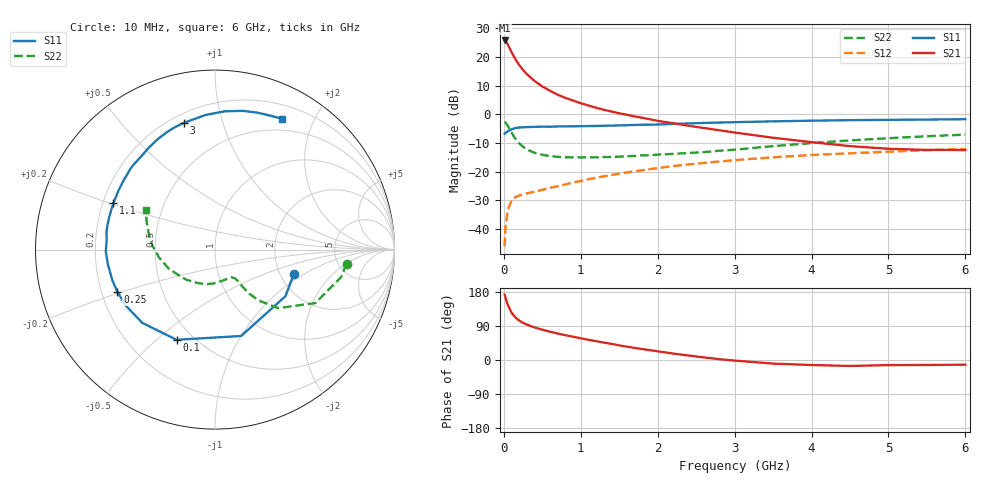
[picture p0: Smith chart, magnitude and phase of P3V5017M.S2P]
! SIEMENS Small Signal Semiconductors
! BFP181
! Si NPN RF Bipolar Junction Transistor in SOT143
! VCE = 0.5 V  IC = 17 mA
! Common Emitter S-Parameters:  March  1996
# GHz  S  MA  R  50
!  f  S11  S21  S12  S22
! GHz  MAG  ANG  MAG  ANG  MAG  ANG  MAG  ANG
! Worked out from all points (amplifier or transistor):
!   36 points, 10 MHz to 6 GHz, reference 50 ohm
!   highest |S21| = 25.7 dB at 10 MHz (marker M1)
!   |S21| within 3 dB of that: start of sweep to 80.39 MHz
!   unconditionally stable (mu >= 1): start of sweep to 19.89 MHz; 189.2 MHz to end of sweep
!   at 250 MHz: K = 1.24, MAG = 18.7 dB, |S12| = -28.0 dB
!   at 1.4 GHz: K = 2.92, MAG = 3.5 dB, |S12| = -21.2 dB
!   at 6 GHz: K = 2.55, MAG = -7.1 dB, |S12| = -12.1 dB
!   S11 on the Smith chart (normalised r, x): 10 MHz: 2.37, -0.82; 100 MHz: 0.41, -0.58; 250 MHz: 0.27, -0.19; 1.1 GHz: 0.24, +0.21; 3 GHz: 0.25, +0.75; 6 GHz: 0.36, +1.58
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0.01  0.4597 -17.2  19.38 172.6  0.005 73.5  0.737 -6.1
0.02  0.4706 -33.5  19.1 165.4  0.0101 71.9  0.7191 -12.3
0.05  0.5029 -73.2  16.64 146.1  0.0211 61.1  0.6342 -28.0
0.1  0.5463 -113.1  12.11 125.0  0.0312 43.9  0.4797 -42.8
0.15  0.5751 -134.8  9.129 112.2  0.0357 37.5  0.3731 -49.4
0.2  0.5872 -148.0  7.222 104.1  0.0382 34.8  0.3116 -52.1
0.25  0.5927 -156.6  5.902 98.0  0.0399 33.6  0.2709 -53.0
0.3  0.5969 -163.2  4.988 93.4  0.0417 34.2  0.243 -53.7
0.4  0.6024 -172.1  3.804 85.9  0.0446 35.8  0.2121 -54.2
0.5  0.6086 -179.0  3.054 80.0  0.0481 37.2  0.1961 -55.2
0.6  0.6055 175.5  2.566 74.7  0.0521 39.6  0.1864 -56.9
0.7  0.6127 170.6  2.194 69.9  0.0557 41.5  0.1806 -59.1
0.9  0.6167 162.9  1.733 61.4  0.0644 43.7  0.1777 -64.3
1.1  0.6222 155.4  1.418 53.3  0.0735 45.3  0.1768 -70.6
1.5  0.6391 142.7  1.039 38.6  0.0917 45.7  0.1819 -84.3
1.8  0.6555 134.0  0.867 28.8  0.1056 44.8  0.1918 -95.3
2.2  0.6769 123.2  0.698 17.0  0.1244 41.8  0.2035 -111.4
3  0.7271 103.9  0.48 -1.6  0.1583 34.8  0.241 -141.1
3.5  0.7519 94.0  0.389 -9.5  0.1773 29.8  0.2777 -157.0
4.5  0.7883 78.7  0.278 -15.7  0.2084 19.5  0.3501 176.3
5.5  0.8075 67.5  0.239 -13.1  0.2363 10.2  0.4138 157.3
6  0.8197 62.8  0.238 -12.3  0.2473 5.3  0.4411 150.0
